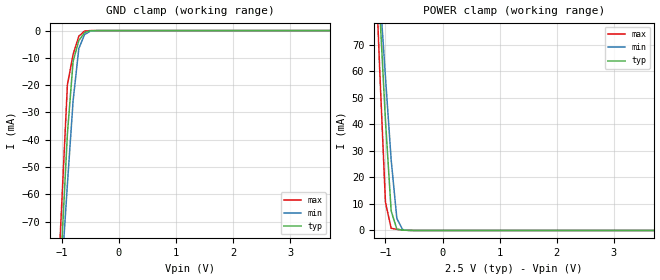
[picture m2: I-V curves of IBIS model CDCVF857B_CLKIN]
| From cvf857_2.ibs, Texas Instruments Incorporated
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|   Diff. Receiver Input MODEL update 8/2003
[Model]   CDCVF857B_CLKIN
Model_type   Input
| Signals   CLK, CLK-, FBIN, FBIN-
Vinl = 1.05V
Vinh = 1.45V
| variable   typ   min   max
C_comp   2.0pF   1.5pF   2.5pF
[Temperature Range]   40.0   105   0
[Voltage range]   2.5V   2.3V   2.7V
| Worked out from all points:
|   GND clamp passes 1 mA (typ) near -0.61 V on its own axis
|   POWER clamp passes 1 mA (typ) near -0.81 V on its own axis
[GND Clamp]
|   40C:2.5V:nominal   105C:2.3V:weak   0C:2.7V:strong
|   Voltage   I(typ)   I(min)   I(max)
-2.7V     -786.9mA   -633.2mA   -974.4mA
-1.1V     -120.2mA   -120.3mA   -107.8mA
-900mV    -37.83mA   -56.32mA   -19.87mA
-800mV    -11.23mA   -25.66mA   -8.694mA
-700mV    -3.681mA   -6.562mA   -2.076mA
-600mV    -729.2uA   -1.486mA   -173.8uA
-500mV    -74.5uA    -243.8uA   -5.751uA
-300mV    -209.7nA   -2.647uA   -734.5pA
5.4V      337.6pA    1.637nA    302.1pA
[POWER Clamp]
|   40C:2.5V:nominal  105C:2.3V:weak   0C:2.7V:strong
|   Voltage   I(typ)   I(min)   I(max)
-2.9V     833mA      666.9mA    1.035A
-1.2V     124.6mA    122.1mA    114.4mA
-1.1V     82.98mA    90.02mA    60.32mA
-1V       41.56mA    58.01mA    10.66mA
-900mV    7.386mA    26.7mA     830.6uA
-800mV    497uA      4.497mA    428.8uA
-700mV    137.9uA    356.4uA    187.5uA
-400mV    675.3nA    1.512uA    268.6nA
5.4V      0A         0A         0A
